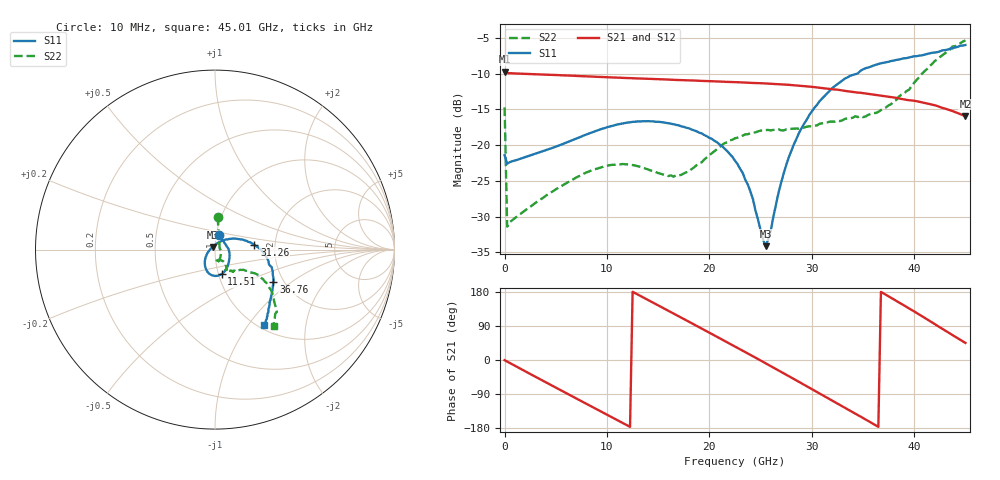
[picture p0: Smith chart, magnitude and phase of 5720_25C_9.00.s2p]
! Device:  ADRF5720
! Description: 0.5dB LSB GaAs MMIC 6-bit Digital Attenuator
! Frequency:  0.000009 -  40 GHz
! Ports:
!	RF1	= Port 1
!	RF2	= Port 2
! Vdd:  3.3 Volt
! Vss:  -3.3 Volt
! Control:  0/3.3 Volt
! State:  9.00 dB attenuation
! Data:  The device was measured using G-S-G Probes on a matrix board.
!  Data was collected using an calibrated 4 port network analyzer.
!  The reference plane for this measurement is at the launchers.
! Note:  Analog Devices supplies this data as a sample of measured data
!  for this product.  Your particular data for this product may vary.
!  Data was taken at 25 degrees C.
!  Analog Devices reserves the right to change this data at anytime.
# GHZ S DB R 45.0
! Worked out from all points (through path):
!   181 points, 10 MHz to 45.01 GHz, reference 45 ohm
!   highest |S21| = -9.76 dB at 10 MHz (marker M1); lowest = -15.9 dB at 45.01 GHz (marker M2)
!   group delay of S21, straight-line fit = 41.3 ps
!   lowest |S11| = -34.1 dB at 25.51 GHz (marker M3), VSWR 1.04, Z = 43.8 + j1.26 ohm
!   |S11| at or under -10 dB: start of sweep to 34.47 GHz
!   |S22| runs from -31.4 to -5.4 dB; largest |S21 - S12| = 0.0004
!   S11 on the Smith chart (normalised r, x): 10 MHz: 1.03, +0.17; 11.51 GHz: 1.03, -0.29; 31.26 GHz: 1.56, +0.09; 36.76 GHz: 1.76, -0.75; 45.01 GHz: 1.07, -1.19
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0.01  -21.42 73.8  -9.76 -0.5  -9.76 -0.5  -14.73 85.4
0.26  -22.61 4.7  -9.94 -4.0  -9.94 -4.0  -31.40 14.8
4.26  -20.61 -30.4  -10.17 -62.1  -10.18 -62.1  -26.87 -45.4
7.76  -18.65 -52.8  -10.38 -112.2  -10.38 -112.2  -23.99 -67.2
11.51  -16.98 -75.2  -10.61 -165.7  -10.61 -165.7  -22.65 -82.8
15.26  -16.78 -95.6  -10.80 140.5  -10.81 140.6  -24.02 -83.2
17.01  -17.24 -104.2  -10.91 115.4  -10.91 115.4  -24.27 -70.9
19.01  -18.27 -113.6  -11.01 86.5  -11.02 86.5  -22.55 -56.9
21.26  -20.18 -125.3  -11.14 53.8  -11.14 53.8  -19.97 -54.5
22.76  -22.67 -137.7  -11.22 31.9  -11.23 31.9  -18.97 -56.2
24.01  -26.48 -154.5  -11.30 13.5  -11.31 13.5  -18.33 -58.8
25.51  -34.13 132.8  -11.39 -8.7  -11.39 -8.7  -17.90 -61.5
27.76  -21.72 43.2  -11.58 -42.6  -11.59 -42.5  -17.78 -60.4
28.76  -18.31 30.6  -11.70 -57.7  -11.70 -57.6  -17.72 -59.7
30.26  -14.80 15.7  -11.90 -80.6  -11.91 -80.6  -17.26 -57.1
31.26  -13.12 7.0  -12.08 -95.9  -12.08 -95.8  -16.86 -55.8
34.01  -10.21 -14.1  -12.58 -137.8  -12.58 -137.8  -16.18 -49.8
36.76  -8.57 -29.3  -13.08 179.7  -13.08 179.7  -15.11 -41.0
37.76  -8.25 -33.8  -13.30 164.1  -13.30 164.2  -14.28 -35.5
41.26  -7.28 -45.4  -14.18 107.4  -14.18 107.5  -9.38 -32.9
43.76  -6.48 -52.4  -15.25 65.6  -15.25 65.6  -6.21 -45.1
45.01  -6.02 -56.9  -15.95 45.1  -15.95 45.2  -5.38 -52.6
